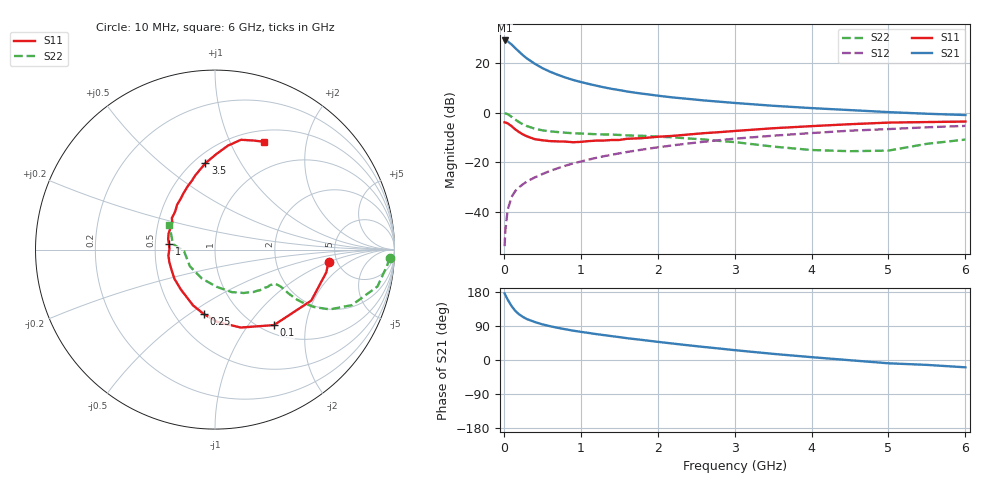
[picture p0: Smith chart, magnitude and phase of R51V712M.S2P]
! SIEMENS Small Signal Semiconductors
! BFR183
! Si NPN RF Bipolar Junction Transistor in SOT23
! VCE = 1.75 V  IC = 12 mA
! Common Emitter S-Parameters:  May  1996
# GHz  S  MA  R  50
!  f  S11  S21  S12  S22
! GHz  MAG  ANG  MAG  ANG  MAG  ANG  MAG  ANG
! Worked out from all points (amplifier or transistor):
!   36 points, 10 MHz to 6 GHz, reference 50 ohm
!   highest |S21| = 28.9 dB at 10 MHz (marker M1)
!   |S21| within 3 dB of that: start of sweep to 146.4 MHz
!   unconditionally stable (mu >= 1): 685.9 MHz to 2.469 GHz
!   at 250 MHz: K = 0.69, MSG = 25.8 dB, |S12| = -28.7 dB
!   at 1.4 GHz: K = 1.06, MAG = 11.8 dB, |S12| = -16.9 dB
!   at 6 GHz: K = 0.91, MSG = 2.2 dB, |S12| = -5.4 dB
!   S11 on the Smith chart (normalised r, x): 10 MHz: 4.27, -0.96; 100 MHz: 1.14, -1.34; 250 MHz: 0.69, -0.57; 1 GHz: 0.59, +0.04; 3.5 GHz: 0.57, +0.72; 6 GHz: 0.64, +1.35
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0.01  0.6363 -6.0  27.82 175.8  0.0021 86.3  0.9739 -2.6
0.02  0.6331 -11.5  27.64 171.3  0.0045 83.1  0.9631 -5.3
0.05  0.6071 -27.9  26.7 159.4  0.0112 77.4  0.9282 -12.8
0.1  0.5337 -52.0  23.15 142.6  0.0203 70.3  0.8226 -22.1
0.15  0.4573 -71.7  19.44 129.3  0.0269 65.3  0.7215 -27.5
0.2  0.4043 -87.8  16.47 120.3  0.032 63.8  0.6382 -30.1
0.25  0.3637 -100.1  13.99 113.4  0.0367 62.6  0.5777 -31.1
0.3  0.3342 -111.4  12.13 108.0  0.0415 63.2  0.5353 -31.4
0.4  0.2927 -130.5  9.547 100.4  0.0499 64.5  0.4753 -30.8
0.5  0.2783 -144.4  7.769 94.1  0.0584 65.1  0.4402 -29.9
0.6  0.2675 -154.5  6.585 89.2  0.0675 66.2  0.42 -29.4
0.7  0.2639 -164.8  5.717 84.9  0.0764 66.6  0.4063 -29.4
0.8  0.2617 -172.7  5.029 81.1  0.0859 66.6  0.3942 -29.5
1  0.2587 172.7  4.089 74.3  0.1042 66.6  0.3793 -30.4
1.1  0.2672 167.6  3.753 71.5  0.1137 66.2  0.3737 -31.5
1.3  0.2742 157.0  3.201 65.7  0.1331 65.0  0.3637 -33.3
1.6  0.2978 143.9  2.647 57.6  0.1617 62.8  0.3491 -37.5
2.2  0.3407 124.4  2.004 43.3  0.2202 57.3  0.3183 -48.0
3.5  0.4845 96.3  1.366 16.2  0.3435 41.4  0.208 -87.1
4.5  0.5838 82.9  1.119 -0.6  0.4331 28.7  0.168 -146.3
5.5  0.6444 70.6  0.946 -12.9  0.5063 16.7  0.2363 172.5
6  0.66 65.5  0.89 -19.3  0.5398 9.1  0.2874 151.9
